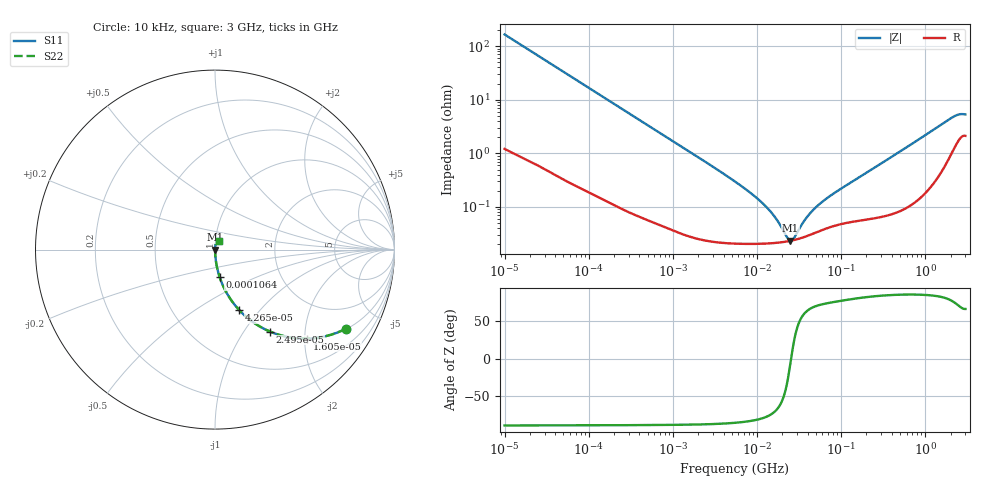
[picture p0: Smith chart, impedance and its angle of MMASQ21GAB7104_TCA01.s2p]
! MMASQ21GAB7104_TCA01  S-PARAMETER MODEL  ( Standard Model )
! Model Generated by TAIYO YUDEN Corporation (http://www.ty-top.com)
! Version 1.0
! TAIYO YUDEN Control No. 220901
! Copyright(c) 2022 TAIYO YUDEN CO.,LTD. All Rights Reserved.
! Product Description (link to TY-COMPAS)
! https://ds.yuden.co.jp/TYCOMPAS/or/detail?pn=MMASQ21GAB7104KTCA01&u=M
! Products Name : Multilayer Ceramic Capacitors
! Characteristics :
!  Capacitance : 0.1 [uF] , Rated Voltage : 250 [V] , TCC : X7R
!  Case Size : 2.0 x 1.25 / 0.079 x 0.049 [mm/inch] , Thickness : 1.25 / 0.049 [mm/inch]
!  (Conditions: Temperature = 25 [degC] , DC Bias Voltage = 0 [V])
! External Node Assignments :
!  1  o---| |---o  2
! GND o---------o GND
! Frequency Range : 10kHz  -  3GHz  [ 401 STEP ]
# MHZ S RI R 50
! Freq[MHz].  S11 Real  S11 Imag  S21 Real  S21 Imag  S12 Real  S12 Imag  S22 Real  S22 Imag
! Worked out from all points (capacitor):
!   401 points, 10 kHz to 3 GHz, reference 50 ohm
!   read as one part in series: C = 96.4 nF near 10.65 kHz
!   lowest |Z| = 23.6 mohm at 24.88 MHz (marker M1)
!   series resonance near 25.45 MHz, so ESL is about 410 pH
!   S11 on the Smith chart (normalised r, x): 10 kHz: 1.02, -3.30; 16.05 kHz: 1.02, -2.06; 24.95 kHz: 1.01, -1.33; 42.65 kHz: 1.01, -0.78; 106.4 kHz: 1.00, -0.31; 3 GHz: 1.04, +0.10
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0.01  0.7295 -0.4405  0.2705 0.4405  0.2705 0.4405  0.7295 -0.4405
0.016047  0.5144 -0.4957  0.4856 0.4957  0.4856 0.4957  0.5144 -0.4957
0.024951  0.3073 -0.457  0.6927 0.457  0.6927 0.457  0.3073 -0.457
0.042645  0.1341 -0.336  0.8659 0.336  0.8659 0.336  0.1341 -0.336
0.082683  0.041 -0.193  0.959 0.193  0.959 0.193  0.041 -0.193
0.106405  0.0257 -0.1527  0.9743 0.1527  0.9743 0.1527  0.0257 -0.1527
0.241531  0.00573 -0.0691  0.9943 0.0691  0.9943 0.0691  0.00573 -0.0691
0.683653  0.00108 -0.0247  0.9989 0.0247  0.9989 0.0247  0.00108 -0.0247
5.477226  0.000216 -0.00297  0.9998 0.00297  0.9998 0.00297  0.000216 -0.00297
9.070798  0.000208 -0.00164  0.9998 0.00164  0.9998 0.00164  0.000208 -0.00164
13.24217  0.000209 -0.000939  0.9998 0.000939  0.9998 0.000939  0.000209 -0.000939
17.04125  0.000215 -0.000551  0.9998 0.000551  0.9998 0.000551  0.000215 -0.000551
22.63272  0.000227 -0.000156  0.9998 0.000156  0.9998 0.000156  0.000227 -0.000156
24.87798  0.000234 -3.01e-05  0.9998 3.01e-05  0.9998 3.01e-05  0.000234 -3.01e-05
27.34599  0.000241 9.54e-05  0.9998 -9.54e-05  0.9998 -9.54e-05  0.000241 9.54e-05
36.31858  0.000275 0.000475  0.9997 -0.000475  0.9997 -0.000475  0.000275 0.000475
45.28751  0.000313 0.000782  0.9997 -0.000782  0.9997 -0.000782  0.000313 0.000782
79.88199  0.000439 0.00169  0.9996 -0.00169  0.9996 -0.00169  0.000439 0.00169
374.4521  0.000773 0.00805  0.9992 -0.00805  0.9992 -0.00805  0.000773 0.00805
2054.98  0.0118 0.044  0.9882 -0.044  0.9882 -0.044  0.0118 0.044
2482.93  0.0193 0.0483  0.9807 -0.0483  0.9807 -0.0483  0.0193 0.0483
3000  0.023 0.0466  0.977 -0.0466  0.977 -0.0466  0.023 0.0466
